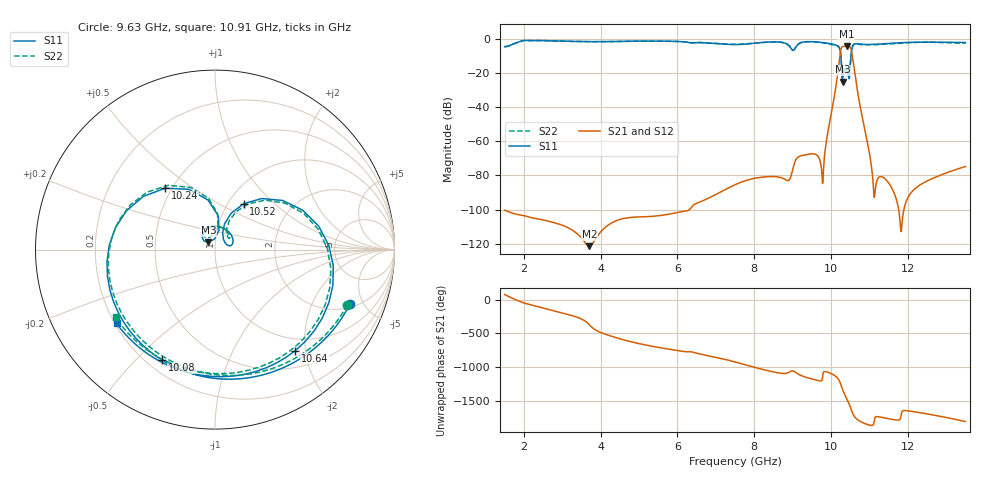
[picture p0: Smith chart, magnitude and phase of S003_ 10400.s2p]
# Hz S DB R 50
! Planar, S50180, , 20.4.1/1
! Date: 14.12.2021 19:09:21
! Data: Format (Calibration Info)
! Freq	S11:dB/Ang(--)	S21:dB/Ang(--)	S12:dB/Ang(--)	S22:dB/Ang(--)
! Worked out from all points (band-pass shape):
!   1201 points, 1.5 GHz to 13.5 GHz, reference 50 ohm
!   highest |S21| = -4.14 dB at 10.41 GHz (marker M1); lowest = -121.5 dB at 3.71 GHz (marker M2)
!   |S21| within 3 dB of the highest: 10.25 GHz to 10.53 GHz (282.2 MHz wide, 2.72 % of centre)
!   lowest |S11| = -25.1 dB at 10.3 GHz (marker M3), VSWR 1.12, Z = 46.3 + j3.82 ohm
!   |S11| at or under -10 dB: 10.26 GHz to 10.52 GHz (266.6 MHz wide, 2.57 % of centre)
!   |S22| runs from -22.5 to -0.9 dB; largest |S21 - S12| = 8.7e-07
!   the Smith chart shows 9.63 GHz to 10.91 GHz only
!   S11 on the Smith chart (normalised r, x): 9.63 GHz: 2.26, -3.97; 10.08 GHz: 0.26, -0.60; 10.24 GHz: 0.46, +0.39; 10.52 GHz: 1.18, +0.66; 10.64 GHz: 0.78, -1.81; 10.91 GHz: 0.21, -0.32
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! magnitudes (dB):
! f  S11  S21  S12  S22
! 1.5 GHz  -4.5  -100.4  -100.4  -4.6
! 3.5 GHz  -1.5  -116.6  -116.6  -1.5
! 3.71 GHz  -1.6  -121.5  -121.5  -1.7
! 5.5 GHz  -1.3  -103.6  -103.6  -1.3
! 7.5 GHz  -3.4  -85.5  -85.5  -3.2
! 8.91 GHz  -4.1  -82.7  -82.7  -4.0
! 9.14 GHz  -3.3  -69.3  -69.3  -3.2
! 9.5 GHz  -1.6  -67.3  -67.3  -1.7
! 9.63 GHz  -1.8  -68.1  -68.1  -2.0
! 9.8 GHz  -2.2  -78.6  -78.6  -2.4
! 10.08 GHz  -3.3  -34.6  -34.6  -3.6
! 10.19 GHz  -4.4  -17.8  -17.8  -4.6
! 10.24 GHz  -7.1  -8.8  -8.8  -7.1
! 10.3 GHz  -25.1  -4.6  -4.6  -22.5
! 10.41 GHz  -18.6  -4.1  -4.1  -18.8
! 10.52 GHz  -10.4  -6.0  -6.0  -10.1
! 10.64 GHz  -2.9  -23.5  -23.5  -3.1
! 10.91 GHz  -3.3  -56.4  -56.4  -3.5
! 11.12 GHz  -3.2  -91.9  -91.9  -3.4
! 11.5 GHz  -2.7  -84.4  -84.4  -3.0
! 12.81 GHz  -2.0  -80.2  -80.2  -2.1
! 13.5 GHz  -2.1  -74.8  -74.8  -2.6
